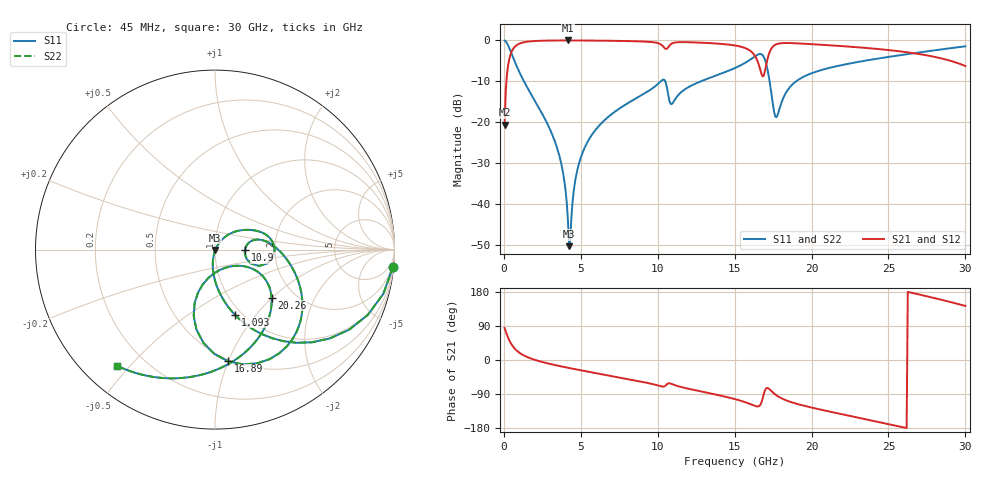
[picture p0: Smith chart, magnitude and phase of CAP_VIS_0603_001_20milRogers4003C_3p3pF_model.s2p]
! S-parameter model data by Modelithics Inc.  support@modelithics.com  813-866-6335  Tampa FL USA
! S-Parameter data specifications:
! Substrate: 20-mil Rogers 4003C, substrate thickness, H=0.508mm, Dielectric constant, Er=3.75
! PCB Mounting Pad Footprint: Pad width, PadW=0.90mm , Pad length, PadL=1.00mm , Pad gap, PadG (edge-to-edge)=1.00mm , Reference planes=3.0mm apart
! Created Wed Nov 18 13:21:45 2015
# hz S ma R 50
! 2 Port Network Data from SP1.SP block
! freq  magS11  angS11  magS21  angS21  magS12  angS12  magS22  angS22
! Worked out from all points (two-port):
!   401 points, 45 MHz to 30 GHz, reference 50 ohm
!   highest |S21| = -0.03 dB at 4.164 GHz (marker M1); lowest = -20.6 dB at 45 MHz (marker M2)
!   |S21| within 3 dB of the highest: 473.9 MHz to 16.16 GHz (15.68 GHz wide, 189 % of centre); 17.26 GHz to 26.44 GHz (9.179 GHz wide, 42 % of centre)
!   lowest |S11| = -50.2 dB at 4.239 GHz (marker M3), VSWR 1.01, Z = 50.2 - j0.246 ohm
!   |S11| at or under -10 dB: 1.304 GHz to 10.19 GHz (8.891 GHz wide, 155 % of centre); 10.48 GHz to 12.8 GHz (2.318 GHz wide, 19.9 % of centre); 17.27 GHz to 18.99 GHz (1.721 GHz wide, 9.49 % of centre)
!   |S22| runs from -50.2 to 0.0 dB; largest |S21 - S12| = 0
!   S11 on the Smith chart (normalised r, x): 45 MHz: 1, -20; 1.093 GHz: 0.93, -0.79; 10.9 GHz: 1.40, -0.00; 16.89 GHz: 0.49, -1.00; 20.26 GHz: 1.54, -0.99; 30 GHz: 0.10, -0.46
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4.5e7  0.9956 -5.6  0.09367 84.4  0.09367 84.4  0.9956 -5.6
4.194375e8  0.7485 -43.6  0.6625 46.4  0.6625 46.4  0.7485 -43.6
1.093425e9  0.3787 -73.1  0.9242 16.8  0.9242 16.8  0.3787 -73.1
3.414938e9  0.05139 -101.6  0.9961 -14.2  0.9961 -14.2  0.05139 -101.6
3.864262e9  0.02303 -101.9  0.9969 -18.1  0.9969 -18.1  0.02303 -101.9
4.163812e9  0.00629 -86.1  0.997 -20.6  0.997 -20.6  0.00629 -86.1
4.2387e9  0.003082 -52.7  0.997 -21.2  0.997 -21.2  0.003082 -52.7
4.688025e9  0.02204 58.0  0.9966 -24.8  0.9966 -24.8  0.02204 58.0
5.062462e9  0.04026 58.2  0.9958 -27.7  0.9958 -27.7  0.04026 58.2
6.560212e9  0.1069 49.1  0.9902 -39.0  0.9902 -39.0  0.1069 49.1
1.007992e10  0.302 14.8  0.9154 -68.0  0.9154 -68.0  0.302 14.8
1.090369e10  0.1667 -0.5  0.9116 -63.3  0.9116 -63.3  0.1667 -0.5
1.50225e10  0.46 -15.8  0.8659 -103.2  0.8659 -103.2  0.46 -15.8
1.629559e10  0.633 -42.4  0.6552 -120.8  0.6552 -120.8  0.633 -42.4
1.689469e10  0.6271 -83.2  0.3727 -89.5  0.3727 -89.5  0.6271 -83.2
1.719424e10  0.3867 -107.9  0.6512 -75.0  0.6512 -75.0  0.3867 -107.9
1.771845e10  0.1154 -63.1  0.8968 -93.2  0.8968 -93.2  0.1154 -63.1
1.86171e10  0.2723 -27.6  0.9269 -110.4  0.9269 -110.4  0.2723 -27.6
2.003996e10  0.3991 -38.4  0.8978 -125.9  0.8978 -125.9  0.3991 -38.4
2.026462e10  0.4129 -40.3  0.8925 -128.0  0.8925 -128.0  0.4129 -40.3
2.505742e10  0.6302 -80.8  0.7594 -169.5  0.7594 -169.5  0.6302 -80.8
3e10  0.8465 -130.2  0.4854 142.7  0.4854 142.7  0.8465 -130.2
